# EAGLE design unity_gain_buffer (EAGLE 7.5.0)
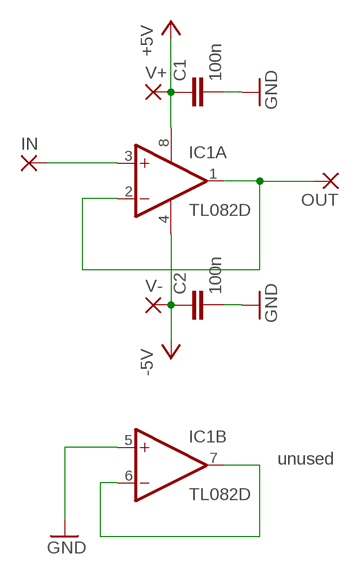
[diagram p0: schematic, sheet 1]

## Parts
C1  100n  C-EUC0805  [C0805]
C2  100n  C-EUC0805  [C0805]
IC1  TL082D  [SO08]
IN  SMD2  [SMD1,27-2,54]
OUT  SMD2  [SMD1,27-2,54]
V+  SMD2  [SMD1,27-2,54]
V-  SMD2  [SMD1,27-2,54]

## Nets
+5V: C1.1 IC1.8(P:V+) V+.1(P)
-5V: C2.1 IC1.4(P:V-) V-.1(P)
GND: C1.2 C2.2 IC1.5(B:+IN)
IN: IC1.3(A:+IN) IN.1(P)
N$3: IC1.6(B:-IN) IC1.7(B:OUT)
OUT: IC1.1(A:OUT) IC1.2(A:-IN) OUT.1(P)

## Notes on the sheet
- unused

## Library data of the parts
C1 C2 = rcl:C-EU: CAPACITOR, European symbol
IC1 = linear:TL082: OP AMP Data sheet; DATA_SHEET: <a href="http://www.ti.com/lit/ds/symlink/tl084a.pdf"> Data sheet </a>
IN OUT V+ V- = wirepad:SMD2: SMD PAD

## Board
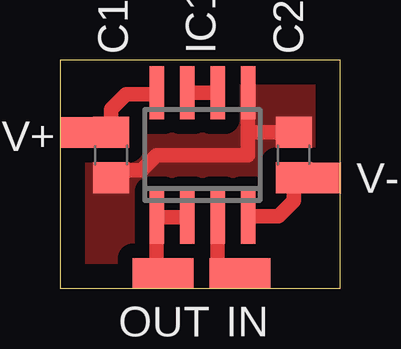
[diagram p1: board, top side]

Size 11.7 x 9.5 mm. Coordinates in mm from the lower left corner, seen from the top.
Outline: 0,0 11.7,0 11.7,9.5 0,9.5 0,0
Copper layers (1*16): Top 0.035mm / dielectric 1.5mm / Bottom 0.035mm
Design rules "default": minimum track width 10mil, minimum drill 24mil, track to track 8mil, track to pad 8mil, pad to pad 8mil, via to via 8mil, smd to smd 8mil, copper to edge 40mil, drill to drill 8mil, minimum pad ring 10mil, minimum via ring 8mil, stop-mask expansion 4mil, vias tented up to drill 0mil, thermal gap 10mil

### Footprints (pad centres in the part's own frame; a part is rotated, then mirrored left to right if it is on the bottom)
C0805 = smd 1.3 x 1.5: 1 -0.95,0; 2 0.95,0
SO08 = smd 0.6 x 2.2: 1 -1.905,-2.6; 2 -0.635,-2.6; 3 0.635,-2.6; 4 1.905,-2.6; 5 1.905,2.6; 6 0.635,2.6; 7 -0.635,2.6; 8 -1.905,2.6
SMD1,27-2,54 = smd 1.27 x 2.54: 1 0,0

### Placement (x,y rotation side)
C1  2.13,5.54 270 top
C2  9.75,5.54 90 top
IC1  5.94,5.54 0 top
IN  7.5,0.6 90 top
OUT  4.3,0.6 270 top
V+  1.27,6.48 270 top
V-  10.44,4.57 90 top

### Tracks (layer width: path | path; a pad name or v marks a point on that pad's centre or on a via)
+5V
  Top 0.61: IC1.8 3.98,8.08 2.77,8.08 2.13,7.45 C1.1 V+.1
-5V
  Top 0.61: IC1.4 7.91,3 9.12,3 9.75,3.63 C2.1 9.77,4.58 V-.1
GND
  Top 0.61: IC1.5 7.84,6.49 | 7.84,6.49 7.84,5.54 4.04,5.54 3.4,4.91 2.44,4.91 C1.2 | C2.2 7.84,6.49
  pour Top (isolate 0.61, no thermals): -0.41,9.75 12.19,9.75 12.19,-0.41 -0.41,-0.41
IN
  Top 0.61: IC1.3 6.58,0.6 IN.1
N$3
  Top 0.61: IC1.7 IC1.6
OUT
  Top 0.61: IC1.2 IC1.1 4.04,0.86 OUT.1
